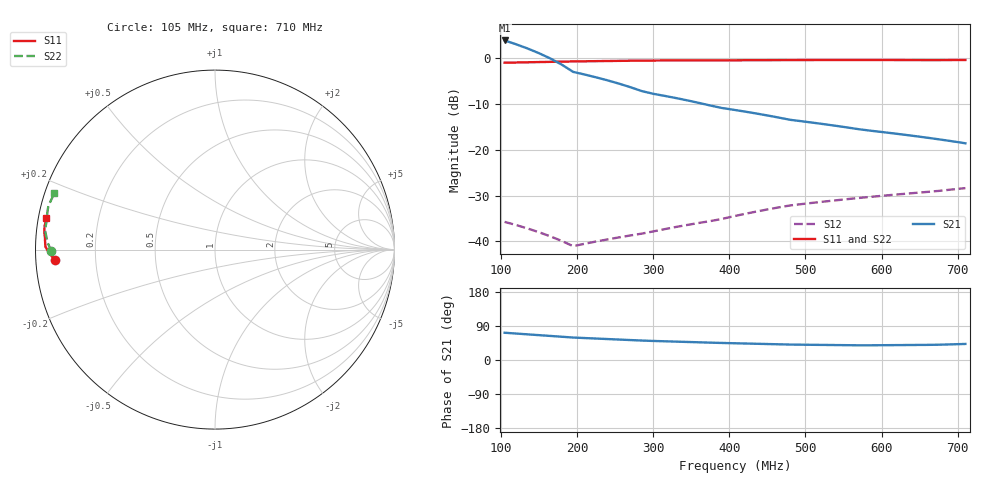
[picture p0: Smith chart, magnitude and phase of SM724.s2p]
!  POLYFET RF DEVICES
!  S PARAMETERS FOR
!  SM724
!  VDS=12.5, IDQ=800MA
# MHZ S MA R 50
! Freq=Mhz Mag[s11] Ang[s11] Mag[s21] Ang[s21] Mag[s12] Ang[s12] Mag[s22] Ang[s22]
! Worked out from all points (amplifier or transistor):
!   42 points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, 105 MHz to 710 MHz, reference 50 ohm
!   highest |S21| = 3.9 dB at 105 MHz (marker M1)
!   |S21| within 3 dB of that: start of sweep to 153 MHz
!   unconditionally stable (mu >= 1): 171.6 MHz to end of sweep
!   at 210 MHz: K = 1.46, MAG = 14.5 dB, |S12| = -40.5 dB
!   at 420 MHz: K = 1.42, MAG = 7.3 dB, |S12| = -34.0 dB
!   at 710 MHz: K = 1.74, MAG = -0.1 dB, |S12| = -28.4 dB
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105  0.8944 -176.2  1.565 71.9  0.01636 -15.1  0.9111 -179.4
120  0.8993 -176.6  1.423 69.8  0.01512 -7.3  0.9146 -179.9
135  0.9042 -177.1  1.28 67.7  0.01387 0.4  0.9182 179.6
150  0.9091 -177.5  1.138 65.6  0.01262 8.2  0.9217 179.1
165  0.914 -178.0  0.9953 63.5  0.01137 16.0  0.9252 178.7
180  0.9189 -178.4  0.8528 61.4  0.01013 23.8  0.9287 178.2
195  0.9238 -178.9  0.7103 59.3  0.00888 31.6  0.9323 177.7
210  0.9271 -179.2  0.665 57.9  0.00943 33.8  0.9356 177.0
255  0.9371 179.8  0.5292 54.0  0.01107 40.5  0.9456 175.0
285  0.9437 179.2  0.4387 51.3  0.01217 45.0  0.9522 173.6
300  0.9453 178.7  0.4097 50.3  0.01286 48.2  0.9531 173.1
315  0.9461 178.3  0.3887 49.4  0.01362 51.8  0.9528 172.8
345  0.9476 177.3  0.3468 47.6  0.01515 59.0  0.9523 172.0
375  0.9491 176.4  0.305 45.8  0.01668 66.2  0.9517 171.3
390  0.9499 176.0  0.2869 45.0  0.01759 69.2  0.9517 170.9
420  0.9518 175.4  0.2622 43.6  0.01997 72.8  0.953 170.0
480  0.9556 174.2  0.2129 40.7  0.02473 80.1  0.9557 168.1
510  0.9565 173.5  0.1979 40.1  0.02643 81.1  0.9569 167.2
570  0.9584 172.2  0.1681 38.8  0.02983 83.2  0.9593 165.6
615  0.9566 171.2  0.1515 39.3  0.03229 85.0  0.9561 164.0
660  0.9544 170.3  0.1357 39.9  0.03474 86.8  0.9522 162.5
710  0.9584 169.3  0.1179 42.4  0.03822 87.7  0.9497 160.6
